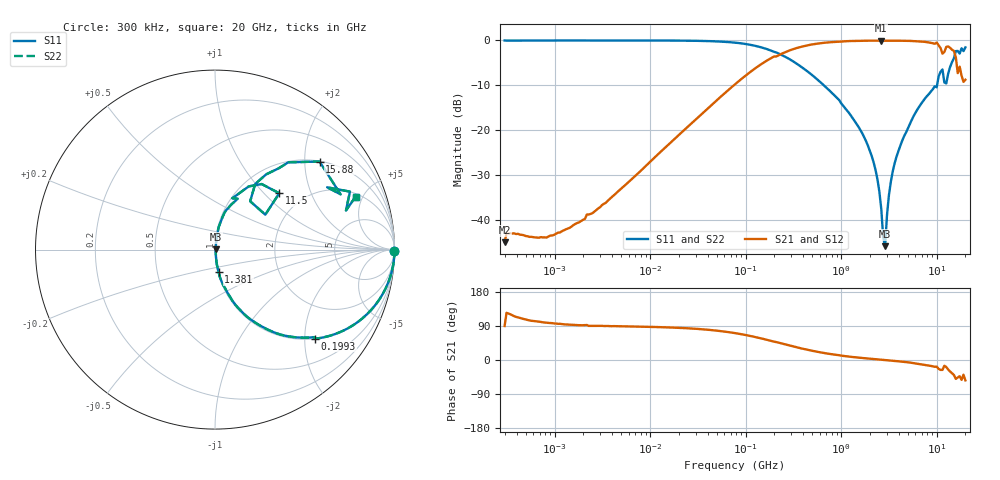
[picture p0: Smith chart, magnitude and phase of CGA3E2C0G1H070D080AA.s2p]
! S-parameter Generated by TDK Corporation
! Copyright(C) 2015 TDK Corporation.
! All Rights Reserved.
! TDK P/N: CGA3E2C0G1H070D080AA (Multilayer Ceramic Chip Capacitors)
! Property: C=7pF
! Size(LxWxT): 1.6x0.8x0.8mm, 0.063x0.031x0.031inches
! Model Type: s2p (Touchstone File Format Version 1.0)
! Frequency: DC=Yes Start=0.3MHz Stop=20000MHz 243points Log-sweep
! Note:
! Model Generated on Jun. 23, 2015
! Hash(MD5):
! Port Assignments:
!  1 ---| |--- 2
! Applicable Conditions:
!  Temperature = 25 degC
!  DC Bias Voltage = 0 V
!  Small Signal Operation
! Terms and conditions regarding TDK Simulation Models
! (1)This simulation model is being provided solely for informational purposes. Please refer to the specifications of the products in terms of detailed characteristics of such products.
! (2)In no event shall TDK Corporation of any of its subsidiaries be liable for any loss or damage arising, directly or indirectly,
!  From any information contained in this simulation model, including, but not limited to loss or damages arising from any inaccuracies, omissions or errors in connection with such information.
! (3)Any and all copyrights on this simulation model are owned by TDK Corporation.
!  Duplication or redistribution of this simulation model without prior written permission from TDK Corporation is prohibited.
! (4)This simulation model is subject to any modification or change without any prior notice.
! (5)Neither TDK Corporation nor any of its subsidiaries shall make any warranty, express or implied,
!  Including but not limited to the correctness, implied warranties of merchantability and fitness for a particular purpose with respect to this simulation models.
! (6)The use of this simulation model shall be deemed to have consented to the terms and conditions hereof.
# MHz S MA R 50
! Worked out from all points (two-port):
!   242 points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, 300 kHz to 20 GHz, reference 50 ohm
!   highest |S21| = -0.04 dB at 2.632 GHz (marker M1); lowest = -44.8 dB at 300 kHz (marker M2)
!   |S21| within 3 dB of the highest: 234.4 MHz to 15.52 GHz (15.29 GHz wide, 194 % of centre)
!   lowest |S11| = -45.7 dB at 2.886 GHz (marker M3), VSWR 1.01, Z = 50.4 + j0.274 ohm
!   |S11| at or under -10 dB: 662.1 MHz to 10.1 GHz (9.435 GHz wide, 175 % of centre)
!   |S22| runs from -45.7 to 0.0 dB; largest |S21 - S12| = 5.4e-14
!   S11 on the Smith chart (normalised r, x): 300 kHz: open; 199.3 MHz: 1.00, -2.25; 1.381 GHz: 1.01, -0.26; 11.5 GHz: 1.51, +1.23; 15.88 GHz: 1.01, +2.36; 20 GHz: 2.23, +4.41
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0.3  1 -0.3  0.00573 89.7  0.00573 89.7  1 -0.3
1.985118  0.9995 -0.6  0.01016 91.7  0.01016 91.7  0.9995 -0.6
12.54397  0.9984 -3.2  0.05634 86.8  0.05634 86.8  0.9984 -3.2
79.26541  0.943 -19.4  0.3327 70.6  0.3327 70.6  0.943 -19.4
199.2545  0.7467 -41.7  0.6647 48.3  0.6647 48.3  0.7467 -41.7
500.8786  0.4101 -64.7  0.9045 24.2  0.9045 24.2  0.4101 -64.7
1380.668  0.1279 -81.1  0.9883 7.3  0.9883 7.3  0.1279 -81.1
2090.428  0.05206 -82.8  0.9948 3.0  0.9948 3.0  0.05206 -82.8
2632.185  0.01346 -72.2  0.996 0.7  0.996 0.7  0.01346 -72.2
2756.339  0.006497 -50.3  0.9959 0.3  0.9959 0.3  0.006497 -50.3
2886.349  0.005182 31.6  0.9956 -0.2  0.9956 -0.2  0.005182 31.6
3165.055  0.01904 75.8  0.9955 -1.1  0.9955 -1.1  0.01904 75.8
3634.376  0.04327 81.3  0.9944 -2.5  0.9944 -2.5  0.04327 81.3
4576.263  0.08699 81.2  0.9904 -5.0  0.9904 -5.0  0.08699 81.2
10018.13  0.3018 71.4  0.947 -17.6  0.947 -17.6  0.3018 71.4
11503.64  0.4761 41.2  0.7147 -26.1  0.7147 -26.1  0.4761 41.2
12046.24  0.3413 34.8  0.7449 -15.1  0.7449 -15.1  0.3413 34.8
13209.43  0.4282 58.5  0.8581 -25.2  0.8581 -25.2  0.4282 58.5
15883.6  0.7614 40.1  0.6483 -49.9  0.6483 -49.9  0.7614 40.1
16632.79  0.7644 23.8  0.4335 -46.1  0.4335 -46.1  0.7644 23.8
17417.32  0.7148 29.1  0.5113 -42.8  0.5113 -42.8  0.7148 29.1
20000  0.8374 20.6  0.366 -53.8  0.366 -53.8  0.8374 20.6
